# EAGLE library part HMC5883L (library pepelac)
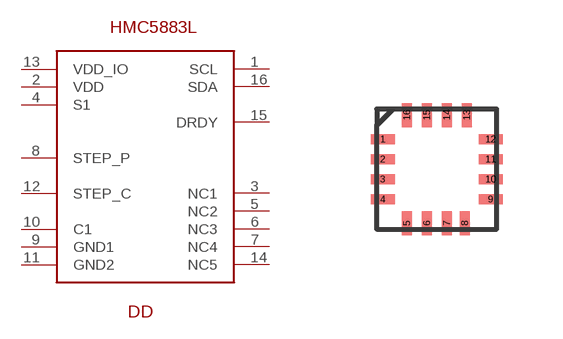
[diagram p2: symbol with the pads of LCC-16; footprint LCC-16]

Designator prefix DD

## HMC5883L  [LCC-16]
1  SCL
2  VDD
3  NC1
4  S1
5  NC2
6  NC3
7  NC4
8  STEP_P
9  GND1
10  C1
11  GND2
12  STEP_C
13  VDD_IO
14  NC5
15  DRDY
16  SDA

## Footprint LCC-16 (pad centres in mm)
LEADLESS CERAMIC CHIP CARRIER
smd 0.6 x 0.25: 1 -1.35,0.85; 2 -1.35,0.35; 3 -1.35,-0.15; 4 -1.35,-0.65; 9 1.35,-0.65; 10 1.35,-0.15; 11 1.35,0.35; 12 1.35,0.85
smd 0.25 x 0.6: 5 -0.75,-1.25; 6 -0.25,-1.25; 7 0.25,-1.25; 8 0.7,-1.25; 13 0.75,1.45; 14 0.25,1.45; 15 -0.25,1.45; 16 -0.75,1.45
